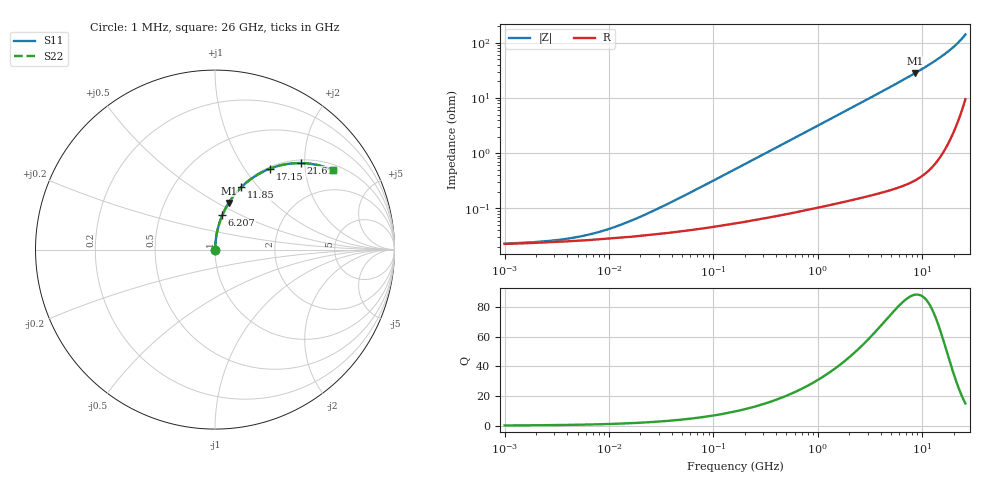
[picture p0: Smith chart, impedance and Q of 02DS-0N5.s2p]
# MHz S MA R 50
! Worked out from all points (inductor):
!   221 points, 1 MHz to 26 GHz, reference 50 ohm
!   read as one part in series: L = 500 pH near 33.51 MHz
!   highest Q = 88.1 at 8.577 GHz (marker M1), where L = 524 pH
!   S11 on the Smith chart (normalised r, x): 1 MHz: 1.00, +0.00; 6.207 GHz: 1.00, +0.40; 11.85 GHz: 1.01, +0.82; 17.15 GHz: 1.03, +1.32; 21.61 GHz: 1.07, +1.92; 26 GHz: 1.19, +2.83
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1  0.0002281 7.9  0.9998 -0.0  0.9998 -0.0  0.0002281 7.9
2.63894  0.000256 18.9  0.9998 -0.0  0.9998 -0.0  0.000256 18.9
3.81921  0.000278 25.6  0.9997 -0.0  0.9997 -0.0  0.000278 25.6
5.52737  0.0003135 33.6  0.9997 -0.0  0.9997 -0.0  0.0003135 33.6
7.9995  0.0003714 42.6  0.9997 -0.0  0.9997 -0.0  0.0003714 42.6
12.1248  0.0004789 52.6  0.9997 -0.0  0.9997 -0.0  0.0004789 52.6
18.3776  0.0006558 61.6  0.9997 -0.0  0.9997 -0.0  0.0006558 61.6
30.5518  0.001019 70.2  0.9997 -0.1  0.9997 -0.1  0.001019 70.2
61.1023  0.001961 78.0  0.9996 -0.1  0.9996 -0.1  0.001961 78.0
168.871  0.00533 83.9  0.9994 -0.3  0.9994 -0.3  0.00533 83.9
891.261  0.02799 86.4  0.9986 -1.6  0.9986 -1.6  0.02799 86.4
2351.98  0.07385 84.6  0.9958 -4.2  0.9958 -4.2  0.07385 84.6
4926.33  0.155 80.3  0.9858 -8.9  0.9858 -8.9  0.155 80.3
6206.74  0.1955 78.0  0.9783 -11.3  0.9783 -11.3  0.1955 78.0
8577.09  0.2711 73.6  0.9595 -15.7  0.9595 -15.7  0.2711 73.6
11852.7  0.3766 67.2  0.9218 -22.1  0.9218 -22.1  0.3766 67.2
14259  0.4543 62.1  0.8842 -27.0  0.8842 -27.0  0.4543 62.1
17153.8  0.5467 55.7  0.8265 -33.1  0.8265 -33.1  0.5467 55.7
18814.7  0.5983 51.9  0.7868 -36.7  0.7868 -36.7  0.5983 51.9
21612.3  0.681 45.1  0.7087 -42.9  0.7087 -42.9  0.681 45.1
23704.9  0.7375 39.8  0.6413 -47.4  0.6413 -47.4  0.7375 39.8
26000  0.7923 33.9  0.5595 -52.2  0.5595 -52.2  0.7923 33.9
